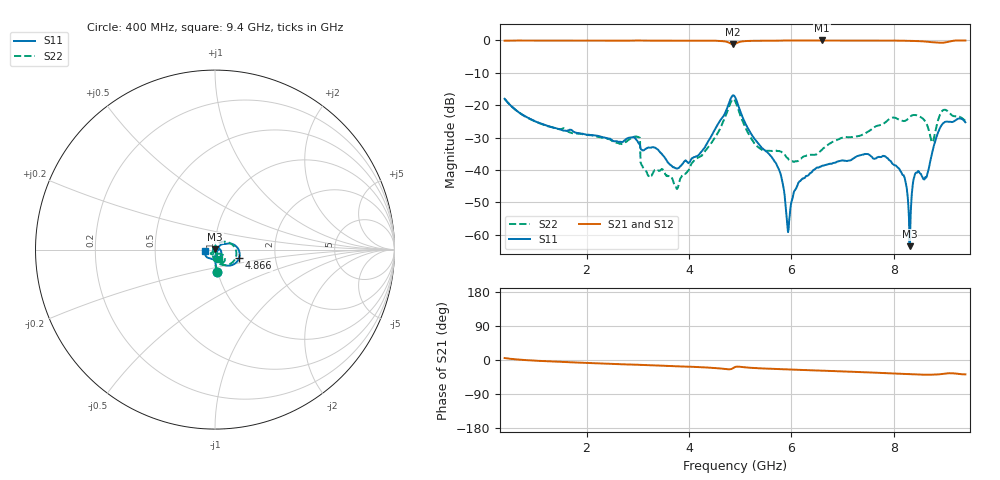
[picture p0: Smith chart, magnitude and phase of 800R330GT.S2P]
!  American Technical Ceramics  Date:  6/19/09
!  One Norden Lane
!  Huntington Station,  NY.  11746-2102
!  Tel:  (631) 622-4700  Fax:  (631) 622-4748
!  Part Number  800R330GT
!  Description: Ultra-low ESR, NPO  Mounting Orientation: Vertical
!  Application: High RF power Filters, Combiners, Matching networks,
!  Antenna, DC block, Bypass and Couplers
# GHZ S DB R 50
! Freq  |S11|  S11 Ph  |S21|  S21 Ph  |S12|  S12 Ph  |S22|  S22 Ph
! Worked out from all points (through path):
!   801 points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, 400 MHz to 9.4 GHz, reference 50 ohm
!   highest |S21| = 0.00 dB at 6.599 GHz (marker M1); lowest = -1.2 dB at 4.866 GHz (marker M2)
!   group delay of S21, straight-line fit = 12.6 ps
!   lowest |S11| = -63.5 dB at 8.309 GHz (marker M3), VSWR 1.00, Z = 50 + j0.0666 ohm
!   |S11| at or under -10 dB: start of sweep to end of sweep
!   |S22| runs from -45.9 to -18.0 dB; largest |S21 - S12| = 0.0028
!   S11 on the Smith chart (normalised r, x): 400 MHz: 0.99, -0.25; 4.866 GHz: 1.30, -0.13; 9.4 GHz: 0.90, -0.01
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0.4  -18.00 -84.3  -0.07 5.2  -0.09 5.2  -18.01 -84.8
1.908  -28.77 -87.5  -0.02 -7.2  -0.03 -7.2  -28.87 -106.7
2.999  -31.18 -76.9  -0.02 -12.7  -0.03 -12.6  -29.76 -134.1
3.111  -33.95 -68.2  -0.03 -13.4  -0.04 -13.3  -39.38 -132.0
3.404  -33.83 -70.2  -0.04 -14.6  -0.05 -14.6  -40.17 -118.6
3.753  -39.52 -33.8  -0.06 -16.6  -0.06 -16.5  -45.52 -164.1
4.023  -37.37 4.8  -0.07 -17.8  -0.08 -17.7  -39.11 147.0
4.866  -16.94 -19.9  -1.23 -21.0  -1.24 -21.0  -18.14 -22.4
4.9  -17.46 -37.0  -1.09 -18.6  -1.09 -18.5  -18.67 -42.6
5.305  -30.86 -72.3  -0.10 -21.4  -0.11 -21.4  -32.21 -100.8
5.744  -39.34 -75.0  -0.06 -23.8  -0.06 -23.7  -34.14 -100.5
5.935  -59.20 -26.8  -0.01 -24.9  -0.02 -24.8  -36.41 -107.0
6.408  -40.58 60.4  -0.03 -27.3  -0.03 -27.2  -35.32 -81.3
6.599  -38.78 62.0  0.00 -28.1  0.00 -28.0  -33.75 -69.1
7.904  -36.84 -44.1  -0.01 -35.3  -0.01 -35.2  -24.41 -65.6
8.196  -41.64 116.7  -0.10 -36.7  -0.09 -36.6  -24.89 -74.7
8.309  -63.52 93.5  -0.12 -37.3  -0.11 -37.2  -23.74 -70.4
8.421  -41.05 149.0  -0.17 -37.9  -0.16 -37.8  -23.05 -79.5
8.624  -42.13 70.8  -0.35 -39.0  -0.34 -38.9  -25.24 -94.7
8.759  -33.96 28.6  -0.53 -38.6  -0.53 -38.6  -31.42 -63.1
8.916  -26.65 -44.4  -0.71 -37.3  -0.70 -37.2  -22.48 -42.5
9.4  -25.27 -174.7  -0.01 -38.0  -0.01 -37.9  -24.77 -67.0
